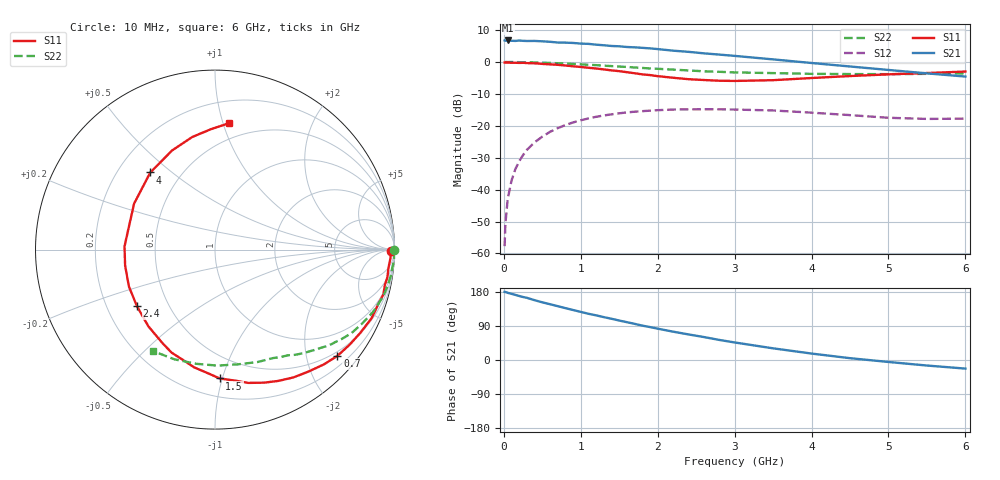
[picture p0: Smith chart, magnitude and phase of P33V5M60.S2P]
! SIEMENS Small Signal Semiconductors
! BFP181
! Si NPN RF Bipolar Junction Transistor in SOT143
! VCE = 3.5 V  IC = 0.6 mA
! Common Emitter S-Parameters:  March  1996
# GHz  S  MA  R  50
!  f  S11  S21  S12  S22
! GHz  MAG  ANG  MAG  ANG  MAG  ANG  MAG  ANG
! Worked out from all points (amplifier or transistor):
!   36 points, 10 MHz to 6 GHz, reference 50 ohm
!   highest |S21| = 6.7 dB at 50 MHz (marker M1)
!   |S21| within 3 dB of that: start of sweep to 2.12 GHz
!   unconditionally stable (mu >= 1): 3.653 GHz to end of sweep
!   at 250 MHz: K = 0.07, MSG = 17.9 dB, |S12| = -29.2 dB
!   at 1.4 GHz: K = 0.44, MSG = 10.7 dB, |S12| = -16.4 dB
!   at 6 GHz: K = 1.40, MAG = 2.8 dB, |S12| = -17.8 dB
!   S11 on the Smith chart (normalised r, x): 10 MHz: 74, -36; 700 MHz: 0.41, -2.62; 1.5 GHz: 0.33, -0.98; 2.4 GHz: 0.33, -0.29; 4 GHz: 0.34, +0.42; 6 GHz: 0.37, +1.05
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0.01  0.9784 -0.6  2.172 179.7  0.0013 80.9  0.9996 -0.2
0.02  0.9781 -1.3  2.15 179.6  0.0029 87.7  0.9996 -0.6
0.05  0.979 -2.7  2.174 177.3  0.0071 90.4  0.9969 -1.4
0.1  0.9719 -5.9  2.15 174.6  0.0139 84.4  0.9987 -2.8
0.15  0.9727 -9.1  2.138 171.8  0.021 83.7  0.9963 -4.3
0.25  0.9708 -14.9  2.144 166.2  0.0348 80.1  0.9919 -7.1
0.4  0.9525 -23.6  2.137 157.8  0.0551 73.8  0.9844 -11.2
0.5  0.9332 -29.8  2.107 152.2  0.0676 69.4  0.9764 -14.1
0.7  0.9032 -41.0  2.017 142.1  0.0918 61.7  0.9554 -19.3
0.9  0.8556 -52.7  1.987 131.9  0.1129 53.7  0.9307 -24.2
1.1  0.8117 -64.4  1.922 122.0  0.1305 46.6  0.9039 -29.0
1.5  0.7186 -87.9  1.762 104.1  0.1569 34.1  0.8472 -37.3
1.9  0.6232 -112.7  1.634 86.9  0.1726 23.1  0.7923 -44.6
2.2  0.5661 -131.0  1.504 74.8  0.1797 16.1  0.7595 -49.4
2.4  0.5374 -144.0  1.442 67.5  0.1813 11.5  0.7369 -52.7
2.8  0.5085 -170.0  1.306 53.0  0.1815 4.0  0.7019 -58.6
3  0.5045 178.0  1.246 46.3  0.1797 0.3  0.686 -61.7
3.5  0.5185 150.4  1.098 30.8  0.174 -6.8  0.6695 -69.4
4  0.5608 130.0  0.964 17.0  0.1607 -11.9  0.6519 -78.7
4.5  0.6019 113.4  0.85 4.8  0.147 -15.0  0.6465 -88.9
5.5  0.6714 91.9  0.663 -14.6  0.1282 -11.1  0.6517 -110.2
6  0.7082 83.7  0.591 -22.7  0.1294 -7.6  0.6621 -121.2
